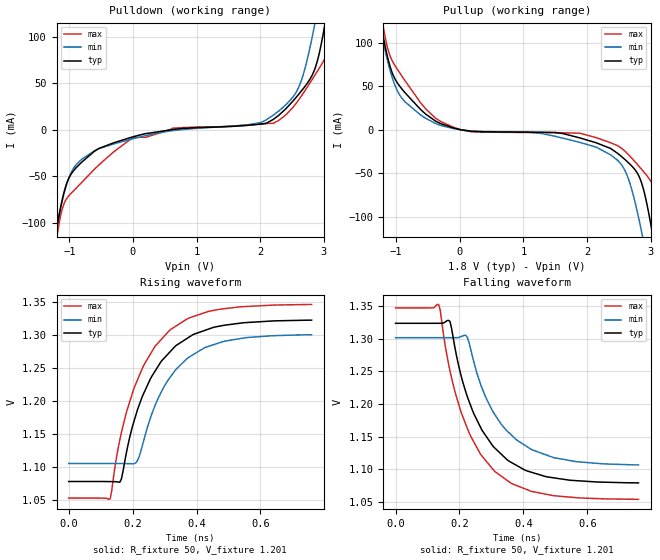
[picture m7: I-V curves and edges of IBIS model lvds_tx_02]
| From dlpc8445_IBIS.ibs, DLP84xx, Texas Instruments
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|   MODEL lvds_tx_02
[Model] lvds_tx_02
Model_type Output
C_comp 1.49p 1.512p 1.443p
Vmeas = 1.2
Vref = 1.2V
Rref = 50
Cref = 0.5pF
[Model Spec]
[Temperature Range]  40 150 -40
[Voltage Range] 1.8 1.62 1.98
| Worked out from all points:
|   slope of the pulldown table from 0 to 0.27 V, typ, clamps not added: 65.1 ohm
|   slope of the pullup table from 0 to 0.27 V, typ, clamps not added: 117 ohm
|   rising waveform, R_fixture 50, V_fixture 1.201: 20-80 % time 133ps typ, 127ps min, 130ps max; typ from 1.08 V to 1.32 V
|   falling waveform, R_fixture 50, V_fixture 1.201: 20-80 % time 130ps typ, 131ps min, 128ps max; typ from 1.32 V to 1.08 V
[Pulldown]
-1.715V   -358.4mA   -310.5mA   -423.2mA
-1.208V   -111mA     -107.1mA   -121.9mA
-1.002V   -51.36mA   -51.05mA   -70.62mA
-536.3mV  -20.18mA   -20.39mA   -37.9mA
18.88mV   -7.253mA   -9.347mA   -8.234mA
2.018V    6.108mA    7.85mA     6.34mA
2.298V    15.79mA    20.4mA     10.24mA
2.62V     39.27mA    47.99mA    33.47mA
2.858V    65.01mA    113.4mA    58.4mA
3.017V    112.9mA    173.7mA    76.21mA
3.16V     175.9mA    231.9mA    109.6mA
3.514V    352.1mA    380.5mA    306mA
[Pullup]
-1.714V   352.1mA    304.9mA    416.6mA
-1.254V   128.2mA    119mA      143.6mA
-1.206V   108.7mA    102.3mA    120.8mA
-1.074V   68.14mA    63.11mA    81.41mA
-910.2mV  47.04mA    36.43mA    61.87mA
-296.9mV  6.914mA    4.875mA    9.374mA
1.501V    -3.154mA   -7.619mA   -3.447mA
2.521V    -29.62mA   -38.39mA   -20.29mA
2.86V     -61.76mA   -118.4mA   -45.75mA
3.034V    -122.2mA   -185.5mA   -64.06mA
3.188V    -193.3mA   -248.5mA   -118.9mA
3.515V    -358.4mA   -386.2mA   -310.8mA
[Ramp]
dV/dt_r .147/133.177p .117/127.859p .176/130.779p
dV/dt_f .147/130.466p .117/132.213p .176/128.106p
[Rising Waveform]
R_fixture = 50
V_fixture = 1.201
V_fixture_min = 1.204
V_fixture_max = 1.2
0s        1.078V     1.106V     1.053V
130ps     1.078V     1.106V     1.052V
165ps     1.082V     1.106V     1.153V
205ps     1.171V     1.106V     1.221V
220ps     1.194V     1.115V     1.238V
255ps     1.233V     1.174V     1.271V
320ps     1.277V     1.238V     1.309V
375ps     1.297V     1.267V     1.326V
485ps     1.315V     1.291V     1.34V
760ps     1.323V     1.301V     1.347V
[Falling Waveform]
R_fixture = 50
V_fixture = 1.201
V_fixture_min = 1.204
V_fixture_max = 1.2
0s        1.324V     1.301V     1.347V
135ps     1.324V     1.301V     1.352V
170ps     1.327V     1.301V     1.251V
205ps     1.243V     1.303V     1.187V
225ps     1.21V      1.302V     1.162V
265ps     1.165V     1.232V     1.124V
310ps     1.133V     1.184V     1.097V
380ps     1.105V     1.144V     1.075V
490ps     1.087V     1.118V     1.06V
760ps     1.079V     1.106V     1.054V
